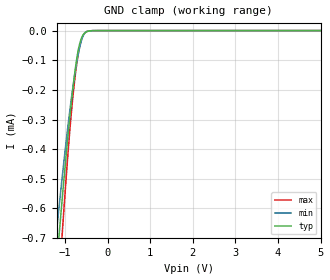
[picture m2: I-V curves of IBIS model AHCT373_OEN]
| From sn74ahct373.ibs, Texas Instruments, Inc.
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[Model]   AHCT373_OEN
Model_type  Input
Vinl = 0.8
Vinh = 2.0
| variable   typ   min   max
C_comp   1.19pF   0.95pF   1.45pF
[Temperature Range]   40   100   -40
| Ambient temperature   25   85   -40
[Voltage range]   5   4.5   5.5
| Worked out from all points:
|   GND clamp passes 1 mA (typ) near -1.32 V on its own axis
[GND Clamp]
| AHCT373_OEN
|   Voltage   I(typ)   I(min)   I(max)
-5V       -9.205mA   -7.488mA   -10.56mA
-1.2V     -794uA     -678.7uA   -975.7uA
-1.155V   -716.2uA   -615.2uA   -876.6uA
-1.115V   -648.3uA   -559.7uA   -789.8uA
-1.075V   -581.7uA   -505.3uA   -704.3uA
-1.04V    -524.6uA   -458.7uA   -630.9uA
-870mV    -267.3uA   -249.7uA   -306.1uA
-750mV    -119.3uA   -128.5uA   -139.1uA
-685mV    -62.05uA   -76.04uA   -74.93uA
-625mV    -29.57uA   -38.55uA   -35.14uA
-495mV    -3.882uA   -3.46uA    -3.425uA
5V        4.223nA    290.1pA    38.48nA
